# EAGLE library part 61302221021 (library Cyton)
WR-PHD 2.54mm Angled Dual Pin Header, 22 Pins =>Code : Con_BTB_PHD_2.54_2_61302221021 Details see: http://katalog.we-online.de/en/em/613_0xx_210_21 Created 2014-05-29, Karrer Zheng 2014 (C) Würth Elektronik
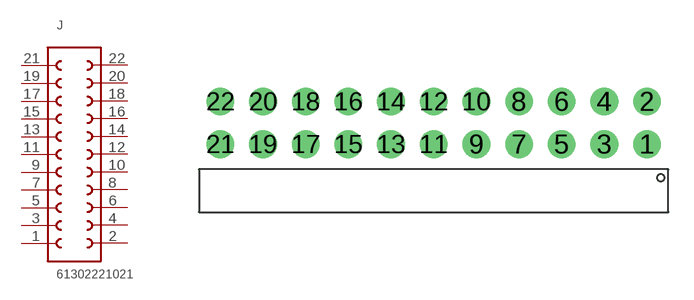
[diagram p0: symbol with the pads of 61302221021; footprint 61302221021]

Designator prefix J

## 61302221021 (AVAILABILITY: Unavailable; DESCRIPTION: WR-PHD 2.54mm Angled Dual Pin Header 22p; MF: Wurth Electronics; MP: 61302221021; PACKAGE: None; PRICE: None)  [61302221021]
1  11  pas
2  12  pas
3  10  pas
4  13  pas
5  9  pas
6  14  pas
7  8  pas
8  15  pas
9  7  pas
10  16  pas
11  6  pas
12  17  pas
13  5  pas
14  18  pas
15  4  pas
16  19  pas
17  3  pas
18  20  pas
19  2  pas
20  21  pas
21  1  pas
22  22  pas

## Footprint 61302221021 (pad centres in mm)
WR-PHD 2.54 mm Angled Dual Pin Header-22 pins, dual row, right angled, gold plating
drill 1.1: 1 12.7,-1.27; 2 12.7,1.27; 3 10.16,-1.27; 4 10.16,1.27; 5 7.62,-1.27; 6 7.62,1.27; 7 5.08,-1.27; 8 5.08,1.27; 9 2.54,-1.27; 10 2.54,1.27; 11 0,-1.27; 12 0,1.27; 13 -2.54,-1.27; 14 -2.54,1.27; 15 -5.08,-1.27; 16 -5.08,1.27; 17 -7.62,-1.27; 18 -7.62,1.27; 19 -10.16,-1.27; 20 -10.16,1.27; 21 -12.7,-1.27; 22 -12.7,1.27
